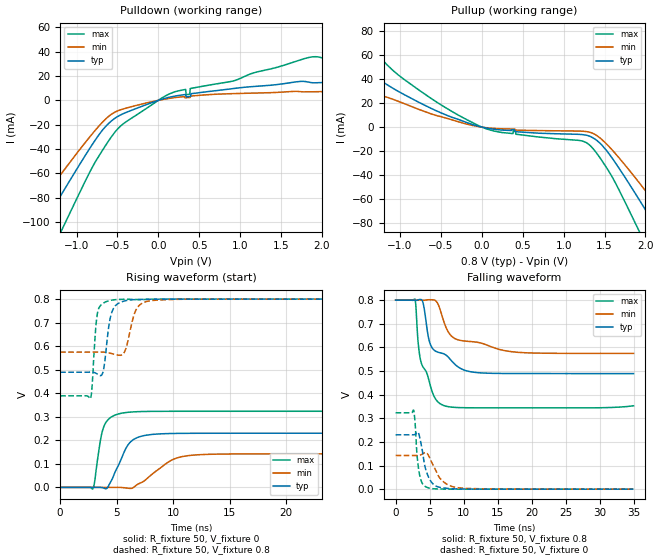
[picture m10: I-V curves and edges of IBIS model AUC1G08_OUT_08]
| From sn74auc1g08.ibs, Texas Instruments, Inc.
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[Model]   AUC1G08_OUT_08
Model_type  Output
Vref =   0
Rref =   2000
Cref =   15p
Vmeas =   0.4
| variable   typ   min   max
C_comp   6.75pF   3.11pF   8.55pF
| C_pullup   5.92pF   3.11pF   8.55pF
| C_pulldown   7.58pF   6.69pF   8.30pF
[Temperature Range]   40   100   -40
| Ambient temperature   25   85   -40
[Voltage range]   0.8   0.8   0.8
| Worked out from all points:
|   slope of the pulldown table from 0 to 0.12 V, typ, clamps not added: 51.5 ohm
|   slope of the pullup table from 0 to 0.12 V, typ, clamps not added: 77.2 ohm
|   rising waveform, R_fixture 50, V_fixture 0: 20-80 % time 1.36ns typ, 2.33ns min, 712ps max; typ from 0 V to 0.23 V
|   falling waveform, R_fixture 50, V_fixture 0.8: 20-80 % time 3.64ns typ, 5.76ns min, 1.96ns max; typ from 0.8 V to 0.489 V
|   rising waveform, R_fixture 50, V_fixture 0.8: 20-80 % time 541ps typ, 735ps min, 350ps max; typ from 0.489 V to 0.8 V
|   falling waveform, R_fixture 50, V_fixture 0: 20-80 % time 1.14ns typ, 1.86ns min, 584ps max; typ from 0.23 V to 0 V
[Pulldown]
| AUC1G08_OUT_08
|   Voltage   I(typ)   I(min)   I(max)
-3.6V     -353.2mA   -290.4mA   -441.2mA
-1.685V   -134mA     -106.3mA   -177.1mA
-1.42V    -103.8mA   -81.62mA   -140.1mA
-1.19V    -77.93mA   -60.65mA   -107.9mA
-605mV    -18.81mA   -13.05mA   -33.04mA
-430mV    -10.99mA   -7.093mA   -19.36mA
115mV     2.243mA    1.381mA    4.628mA
385mV     3.191mA    2.404mA    5.08mA
395mV     3.265mA    3.372mA    9.763mA
1.875V    14.52mA    7.044mA    35.64mA
2.185V    15.03mA    7.402mA    32.01mA
7.2V      28.73mA    13.6mA     59.73mA
[Pullup]
| AUC1G08_OUT_08
|   Voltage   I(typ)   I(min)   I(max)
-3.6V     89.78mA    20.19mA    178.7mA
-3.085V   82.76mA    22.36mA    148.8mA
-1.86V    37.13mA    18.79mA    108mA
-1.55V    45.24mA    12.5mA     83.03mA
-1.21V    37.8mA     25.85mA    55.76mA
-40mV     680.8uA    422.2uA    1.22mA
1.335V    -8.097mA   -4.593mA   -16.14mA
1.875V    -55.34mA   -42.22mA   -80.14mA
1.995V    -68.51mA   -52.69mA   -97.14mA
2.125V    -83mA      -64.29mA   -115.6mA
2.42V     -116.4mA   -91.29mA   -157.4mA
7.2V      -667mA     -555.4mA   -823.9mA
[Ramp]
| AUC1G08_OUT_08
| variable   typ   min   max
dV/dt_r   0.14/1.39E-09   0.09/2.40E-09   0.20/7.16E-10
dV/dt_f   0.19/3.63E-09   0.14/5.75E-09   0.28/2.02E-09
R_load = 50
[Rising Waveform]
| AUC1G08_OUT_08
R_fixture =   50
C_fixture =   0
L_fixture =   0
V_fixture =   0
V_fixture_min = 0
V_fixture_max = 0
|   Time   V(typ)   V(min)   V(max)
0s        3.51nV     13.75nV    219.8pV
2.88ns    86.63uV    -9.572uV   -6.55mV
3.57ns    -44.65uV   11.32uV    202.2mV
3.865ns   -3.357mV   72.12uV    258.4mV
4.215ns   1.085mV    157uV      286.6mV
5.45ns    126.4mV    -481uV     315.2mV
6.945ns   213.9mV    15.48mV    321.8mV
9.775ns   228.8mV    113.8mV    323.3mV
11.57ns   229.8mV    136.3mV    323.3mV
34.99ns   230.1mV    142.6mV    323.3mV
[Falling Waveform]
| AUC1G08_OUT_08
R_fixture =   50
C_fixture =   0
L_fixture =   0
V_fixture =   0.8
V_fixture_min = 0.8
V_fixture_max = 0.8
|   Time   V(typ)   V(min)   V(max)
0s        800mV      800mV      800mV
2.845ns   799.7mV    800mV      804.3mV
3.31ns    801mV      799.9mV    622mV
3.72ns    802.7mV    799.7mV    539.9mV
5.125ns   612mV      801.7mV    436.4mV
6.075ns   581.4mV    791.5mV    374mV
6.9ns     574.7mV    726.7mV    356.1mV
8.71ns    528.6mV    637.5mV    346.1mV
16.1ns    489.7mV    586mV      344.2mV
34.99ns   489.2mV    574.6mV    352.8mV
[Rising Waveform]
| AUC1G08_OUT_08
R_fixture =   50
C_fixture =   0
L_fixture =   0
V_fixture =   0.8
V_fixture_min = 0.8
V_fixture_max = 0.8
|   Time   V(typ)   V(min)   V(max)
0s        489.1mV    574.6mV    388.8mV
2.675ns   489.7mV    574.8mV    377.5mV
2.8ns     489.6mV    574.8mV    414.9mV
3.305ns   480.9mV    575mV      741.9mV
3.81ns    494.8mV    574.6mV    782.3mV
4.36ns    702.4mV    570.7mV    793.3mV
5.6ns     790.7mV    568.9mV    799mV
6.71ns    797.9mV    754.3mV    798mV
7.93ns    799.2mV    792.5mV    799.2mV
34.99ns   800mV      800mV      800mV
[Falling Waveform]
| AUC1G08_OUT_08
R_fixture =   50
C_fixture =   0
L_fixture =   0
V_fixture =   0
V_fixture_min = 0
V_fixture_max = 0
|   Time   V(typ)   V(min)   V(max)
0s        230.1mV    142.7mV    323.4mV
2.65ns    229.9mV    142.5mV    333.8mV
2.85ns    231.6mV    142.4mV    286mV
3.185ns   240.9mV    142.6mV    133.6mV
3.505ns   224.3mV    143.6mV    63.7mV
4.3ns     97.98mV    154.6mV    12.42mV
4.855ns   50.57mV    141.4mV    5.324mV
6.605ns   7.192mV    43.49mV    712.2uV
8.95ns    1.091mV    7.148mV    162.3uV
34.99ns   22.85uV    7.033uV    10.49uV
